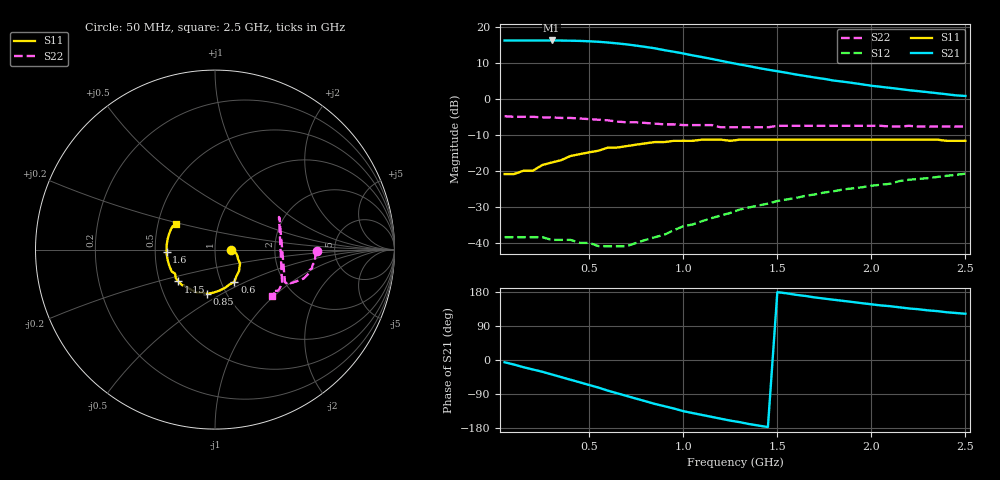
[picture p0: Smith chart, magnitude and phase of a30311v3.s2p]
!	INA-30311	S PARAMETERS
!	Vd = 3 V	LAST UPDATED 1-5-95
# ghz	s ma r 50
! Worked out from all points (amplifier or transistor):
!   50 points, 50 MHz to 2.5 GHz, reference 50 ohm
!   highest |S21| = 16.1 dB at 300 MHz (marker M1)
!   |S21| within 3 dB of that: start of sweep to 935 MHz
!   unconditionally stable (mu >= 1): start of sweep to end of sweep
!   at 450 MHz: K = 5.47, MAG = 17.7 dB, |S12| = -40.0 dB
!   at 1.3 GHz: K = 4.50, MAG = 10.6 dB, |S12| = -30.8 dB
!   at 2.5 GHz: K = 3.99, MAG = 1.8 dB, |S12| = -20.8 dB
!   S11 on the Smith chart (normalised r, x): 50 MHz: 1.20, -0.00; 600 MHz: 1.15, -0.43; 850 MHz: 0.82, -0.43; 1.15 GHz: 0.63, -0.24; 1.6 GHz: 0.58, -0.02; 2.5 GHz: 0.62, +0.19
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0.05  0.09 -1.0  6.4 -6.0  0.012 2.0  0.57 -1.0
0.1  0.09 -2.0  6.39 -12.0  0.012 4.0  0.56 -3.0
0.15  0.1 -3.0  6.39 -19.0  0.012 5.0  0.56 -5.0
0.2  0.1 -6.0  6.4 -25.0  0.012 8.0  0.56 -7.0
0.3  0.13 -16.0  6.41 -38.0  0.011 13.0  0.55 -11.0
0.4  0.16 -29.0  6.36 -52.0  0.011 19.0  0.54 -14.0
0.5  0.18 -42.0  6.24 -66.0  0.01 27.0  0.52 -18.0
0.6  0.21 -59.0  6 -81.0  0.009 40.0  0.5 -20.0
0.7  0.22 -75.0  5.65 -95.0  0.009 57.0  0.47 -23.0
0.8  0.24 -92.0  5.21 -109.0  0.011 74.0  0.46 -24.0
0.85  0.25 -100.0  4.98 -116.0  0.012 81.0  0.45 -24.0
0.9  0.25 -107.0  4.7 -122.0  0.013 86.0  0.44 -24.0
1  0.26 -122.0  4.23 -135.0  0.017 94.0  0.43 -25.0
1.15  0.27 -139.0  3.56 -150.0  0.022 98.0  0.43 -25.0
1.2  0.27 -144.0  3.35 -155.0  0.024 100.0  0.4 26.0
1.3  0.27 -153.0  2.98 -164.0  0.029 100.0  0.4 26.0
1.45  0.27 -166.0  2.52 -177.0  0.035 100.0  0.4 27.0
1.5  0.27 -169.0  2.4 179.0  0.038 101.0  0.42 -27.0
1.6  0.27 -177.0  2.16 172.0  0.042 100.0  0.42 -28.0
1.7  0.27 178.0  1.96 165.0  0.047 100.0  0.42 -29.0
2.1  0.27 159.0  1.41 142.0  0.066 98.0  0.41 -34.0
2.5  0.26 147.0  1.09 122.0  0.091 91.0  0.41 -39.0
